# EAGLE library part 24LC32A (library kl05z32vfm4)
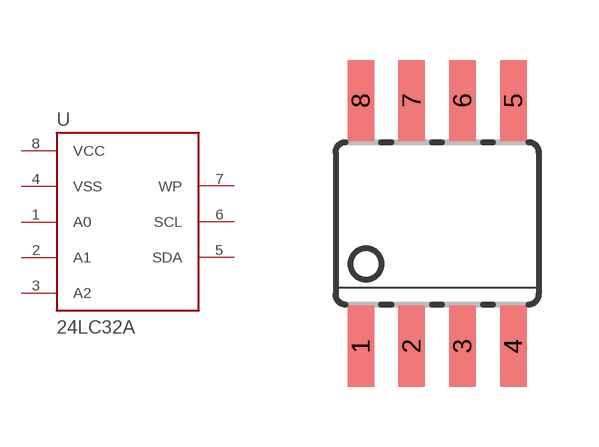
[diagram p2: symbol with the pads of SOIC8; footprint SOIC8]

Designator prefix -

## 24LC32A  [SOIC8]
1  A0
2  A1
3  A2
4  VSS
5  SDA
6  SCL
7  WP
8  VCC

## Footprint SOIC8 (pad centres in mm)
smd 0.66 x 2.032: 1 -1.905,-3.073; 2 -0.635,-3.073; 3 0.635,-3.073; 4 1.905,-3.073; 5 1.905,3.073; 6 0.635,3.073; 7 -0.635,3.073; 8 -1.905,3.073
